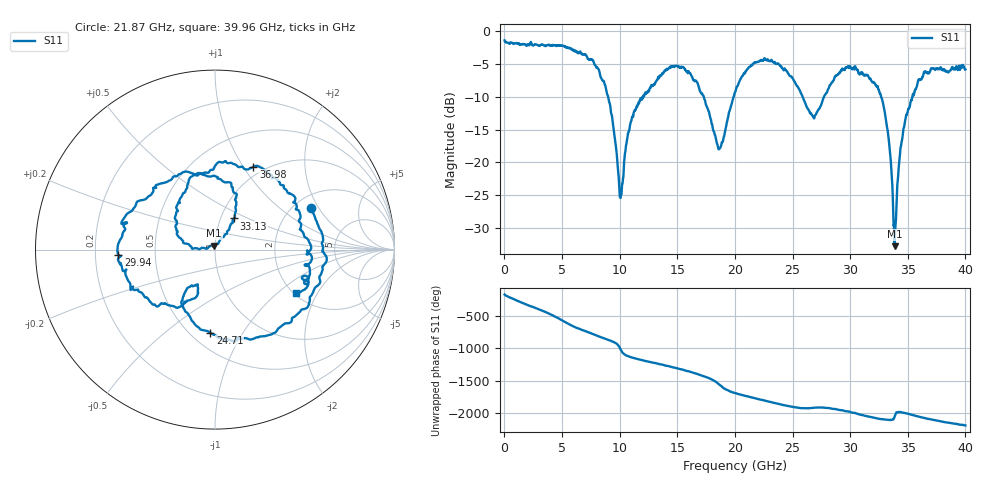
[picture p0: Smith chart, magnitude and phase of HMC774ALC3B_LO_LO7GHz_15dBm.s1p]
! Analog Devices, Inc.
! 1 Analog Way
! Wilmington, MA 01887
! http://www.analog.com
! Date:  2021-09-17 NN
! Board Name:  EV1HMC774ALC3B Revision A with HMC774ALC3B installed
! File Description:  S-Parameters for evaluation board without connectors or board loss de-embedded
! File Generation:  Calibrated Network Analyzer
! Chip Part Number:  HMC774ALC3B
! Chip Description:  MMIC, Double Balanced Mixer
! Chip Frequency:  7 to 34 GHz
! Chip Package:  LCC, 2.9 x 2.9 x 0.8 mm
! Chip State:
!  Temperature:  25C
!  LO Power:  15dBm
! Note:
!  Analog Devices supplies this data as a sample of measured data at the evaluation board
!  ports for this product.  Your particular data for this product may vary.
!  Analog Devices reserves the right to change this data at anytime.
!  All lines below in this file are as is from the Network Analyzer.
!Keysight Technologies,N5245A,MY49151104,A.10.65.16
!Date: Thursday, September 16, 2021 12:20:03
!Correction: S11(Full 1 Port(1))
!S1P File: Measurement: S11:
# Hz S  dB  R 50
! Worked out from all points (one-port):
!   4000 points, 10 MHz to 40 GHz, reference 50 ohm
!   lowest |S11| = -32.8 dB at 33.85 GHz (marker M1), VSWR 1.05, Z = 49.4 + j2.21 ohm
!   |S11| at or under -10 dB: 8.997 GHz to 12.04 GHz (3.038 GHz wide, 28.9 % of centre); 17.31 GHz to 19.89 GHz (2.581 GHz wide, 13.9 % of centre); 32.68 GHz to 35.38 GHz (2.7 GHz wide, 7.93 % of centre)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
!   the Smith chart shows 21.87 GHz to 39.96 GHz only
!   S11 on the Smith chart (normalised r, x): 21.87 GHz: 2.45, +1.71; 24.71 GHz: 0.62, -0.73; 29.94 GHz: 0.30, -0.02; 33.13 GHz: 1.16, +0.42; 36.98 GHz: 0.89, +1.11; 39.96 GHz: 2.05, -1.35
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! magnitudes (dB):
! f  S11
! 10 MHz  -1.4
! 5.01 GHz  -2.2
! 7.58 GHz  -4.3
! 8.62 GHz  -7.6
! 9.31 GHz  -12.7
! 10.01 GHz  -25.3
! 10.18 GHz  -24.0
! 10.78 GHz  -15.2
! 11.42 GHz  -11.8
! 15.01 GHz  -5.3
! 16.73 GHz  -7.8
! 18.61 GHz  -18.0
! 20.01 GHz  -9.3
! 21.87 GHz  -4.7
! 24.71 GHz  -6.6
! 25.01 GHz  -7.2
! 26.86 GHz  -13.3
! 29.94 GHz  -5.4
! 30.01 GHz  -5.3
! 32.29 GHz  -8.4
! 33.13 GHz  -13.8
! 33.45 GHz  -18.3
! 33.85 GHz  -32.8
! 34.43 GHz  -17.3
! 35.01 GHz  -12.2
! 36.98 GHz  -5.9
! 39.96 GHz  -5.8
! 40 GHz  -5.8
